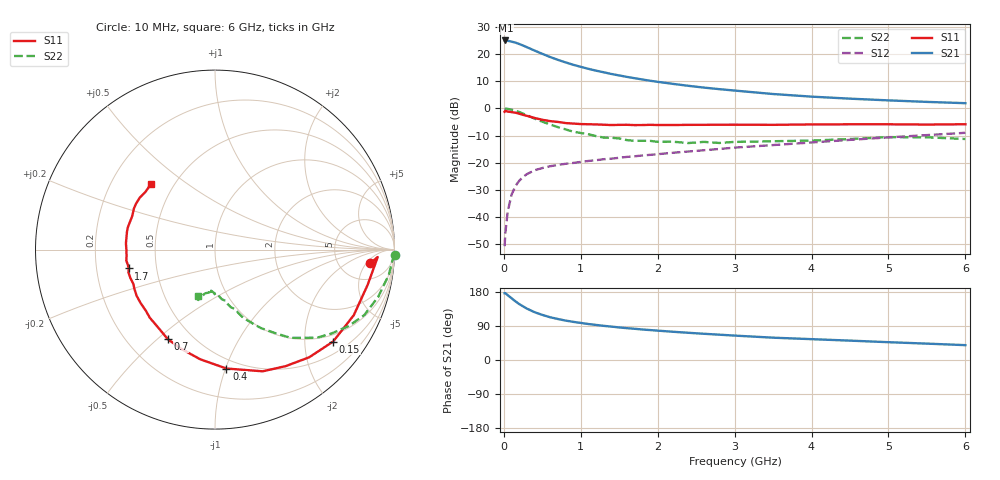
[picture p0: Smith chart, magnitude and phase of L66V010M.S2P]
!  INFINEON TECHNOLOGIES Small Signal Semiconductors
! BFR380L3 , Si-NPN RF-Transistor in TSLP-3-1
!  Vce=6 V,  Ic=10 mA
! Common Emitter S-Parameters:  07. March 2005
#  GHz  S  MA  R  50
! f  S11  S21  S12  S22
! GHz  Mag  Ang  Mag  Ang  Mag  Ang  Mag  Ang
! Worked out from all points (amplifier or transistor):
!   36 points, 10 MHz to 6 GHz, reference 50 ohm
!   highest |S21| = 25.0 dB at 20 MHz (marker M1)
!   |S21| within 3 dB of that: start of sweep to 341.2 MHz
!   unconditionally stable (mu >= 1): 2.713 GHz to 4.593 GHz
!   at 250 MHz: K = 0.21, MSG = 24.2 dB, |S12| = -25.3 dB
!   at 1.4 GHz: K = 0.80, MSG = 15.6 dB, |S12| = -18.5 dB
!   at 6 GHz: K = 0.95, MSG = 5.5 dB, |S12| = -9.0 dB
!   S11 on the Smith chart (normalised r, x): 10 MHz: 10, -6; 150 MHz: 0.80, -2.70; 400 MHz: 0.42, -1.01; 700 MHz: 0.37, -0.54; 1.7 GHz: 0.34, -0.10; 6 GHz: 0.37, +0.37
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0.01  0.868 -5.0  17.76 176.3  0.0029 78.0  1.005 -1.6
0.02  0.9076 -2.6  17.83 176.5  0.0051 82.8  0.9904 -3.4
0.05  0.8729 -13.0  17.53 171.2  0.0125 85.1  0.9788 -8.2
0.1  0.8552 -25.3  16.96 163.0  0.0257 76.9  0.9468 -16.1
0.15  0.8339 -37.9  16.29 155.0  0.037 70.8  0.9083 -23.7
0.2  0.7972 -48.8  15.35 147.6  0.0465 66.5  0.8583 -29.7
0.25  0.7596 -58.7  14.38 141.5  0.0546 61.7  0.7998 -35.8
0.3  0.7283 -68.6  13.38 135.6  0.0616 58.6  0.7502 -40.9
0.4  0.6656 -84.5  11.61 126.1  0.0725 53.5  0.6478 -49.4
0.5  0.6169 -97.6  10.11 119.0  0.0797 50.3  0.5687 -54.6
0.6  0.5833 -109.2  8.847 112.9  0.0859 47.9  0.5062 -59.7
0.7  0.5637 -117.9  7.862 108.3  0.0908 47.0  0.4533 -63.7
0.9  0.5253 -133.8  6.367 100.7  0.0988 46.4  0.373 -70.0
1.1  0.5104 -144.3  5.35 94.9  0.1076 47.0  0.3339 -74.5
1.4  0.4934 -157.2  4.296 88.1  0.1187 48.8  0.2878 -79.4
1.7  0.4923 -167.7  3.594 82.4  0.1311 50.6  0.2531 -85.4
2.2  0.4937 -179.9  2.826 74.5  0.1524 53.2  0.2432 -90.7
2.8  0.5004 168.4  2.262 66.8  0.1788 56.2  0.2309 -98.2
3.5  0.4977 157.8  1.839 58.9  0.211 57.1  0.2483 -102.1
4.5  0.5091 149.8  1.51 51.1  0.2631 59.0  0.2726 -106.0
5.5  0.5036 140.4  1.317 43.2  0.3222 58.0  0.293 -108.9
6  0.5104 134.4  1.247 39.2  0.3551 56.8  0.273 -110.1
